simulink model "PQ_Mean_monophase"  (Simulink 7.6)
settings: Solver=ode15s  StartTime=0.0  StopTime=0.1  RelTol=1e-3
InitFcn:
  | clear all, close all
  | Arms=20;
  | T=1/60;
  | 
  | % charge de la phase C
  | R1=2;
  | 
  | % Charge R, L de la phase B
  | R=1;
  | L=0.1;
StopFcn:
  | close all
  | load PQ_PhaseC.mat
  | subplot 211
  | plot(x(1,:),x(2,:))
  | grid
  | title('Puissance active Phase C')
  | xlabel('temps')
  | 
  | subplot 212
  | plot(x(1,:),x(3,:))
  | title('Puissance réactive Phase C')
  | grid
  | xlabel('temps')
  | 
  | figure
  | 
  | load Moy_PhaseC.mat
  | subplot 211
  | plot(y(1,:),y(2,:))
  | grid
  | title('Moyenne amplitude Phase C')
  | xlabel('temps')
  | axis([0 0.1 0 1100])
  | 
  | subplot 212
  | plot(y(1,:),y(3,:))
  | title('Moyenne phase Phase C')
  | grid
  | xlabel('temps')
undefined symbols (not defined in the file or in its folder): Ts
libraries: powerlib x8, powerlib_extras x2

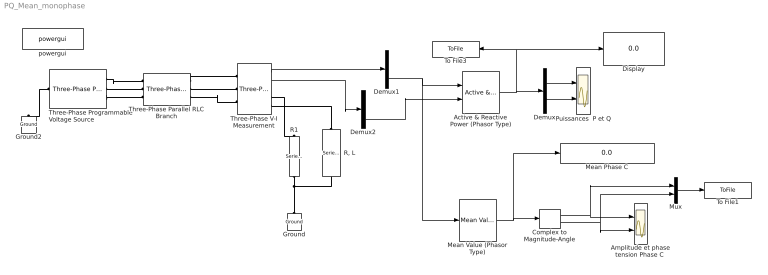
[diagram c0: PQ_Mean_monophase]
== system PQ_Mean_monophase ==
  Active & Reactive Power (Phasor Type) : powerlib_extras/Phasor Library/Active & Reactive Power (Phasor Type)  DialogController=POWERSYS.PowerSysDialog  SystemSampleTime=-1
  "Amplitude et phase tension Phase C " : Scope  NumInputPorts=2
  Complex to Magnitude-Angle : ComplexToMagnitudeAngle
  Demux : Demux  Outputs=2
  Demux1 : Demux  Outputs=3
  Demux2 : Demux  Outputs=3
  Display : Display
  Ground : powerlib/Elements/Ground  DialogController=POWERSYS.PowerSysDialog  PhysicalDomain=powersysdomain  SubClassName=unknown  LeftPortType=p1  RightPortType=p1  LConnTagsString=a
  Ground2 : powerlib/Elements/Ground  DialogController=POWERSYS.PowerSysDialog  PhysicalDomain=powersysdomain  SubClassName=unknown  LeftPortType=p1  RightPortType=p1  LConnTagsString=a
  Mean Phase C : Display
  Mean Value (Phasor Type) : powerlib_extras/Phasor Library/Mean Value (Phasor Type)  DialogController=POWERSYS.PowerSysDialog  SystemSampleTime=-1  Period=1/60
  Mux : Mux  Inputs=2
  Puissances  P et Q : Scope  NumInputPorts=2
  "R, L" : powerlib/Elements/Series RLC Branch  DialogController=POWERSYS.PowerSysDialog  PhysicalDomain=powersysdomain  SubClassName=unknown  LeftPortType=p1  RightPortType=p1  LConnTagsString=__new0  RConnTagsString=__new0  BranchType=RL  Resistance=R  Inductance=L  SetiL0=off  InitialCurrent=0  Capacitance=1e-3  Setx0=off  InitialVoltage=0  Measurements=None
  R1 : powerlib/Elements/Series RLC Branch  DialogController=POWERSYS.PowerSysDialog  PhysicalDomain=powersysdomain  SubClassName=unknown  LeftPortType=p1  RightPortType=p1  LConnTagsString=__new0  RConnTagsString=__new0  BranchType=R  Resistance=R1  Inductance=1e-3  SetiL0=off  InitialCurrent=0  Capacitance=1e-6  Setx0=off  InitialVoltage=0  Measurements=None
  Three-Phase Parallel RLC Branch : powerlib/Elements/Three-Phase Parallel RLC Branch  DialogController=POWERSYS.PowerSysDialog  PhysicalDomain=powersysdomain  SubClassName=unknown  LeftPortType=p1  RightPortType=p1  LConnTagsString=A|B|C  RConnTagsString=A|B|C  BranchType=RLC  Resistance=1  Inductance=1e-3  Capacitance=1e-6  Measurements=None
  Three-Phase Programmable Voltage Source : powerlib/Electrical Sources/Three-Phase Programmable Voltage Source  DialogController=POWERSYS.PowerSysDialog  SystemSampleTime=-1  PositiveSequence="[Arms  0 1/T]"  VariationEntity=Amplitude  VariationType=Step  VariationStep=60  VariationRate=10  VariationMagnitude=0.3  VariationFrequency=2  VariationTiming=[0.02 0.08]  VariationPhaseA=off  Amplitudes=[1 0.8 1.2 1.0]  TimeValues=[0 0.1 0.15 0.2]  HarmonicGeneration=off  HarmonicA="[3 0.2  -25 0]"  HarmonicB=[2 0.15 35 2]  Timing="[0.1  0.2]"
  Three-Phase V-I Measurement : powerlib/Measurements/Three-Phase V-I Measurement  DialogController=POWERSYS.PowerSysDialog  SystemSampleTime=-1  VoltageMeasurement=phase-to-ground  SetLabelV=off  LabelV=Vabc  Vpu=off  VpuLL=off  CurrentMeasurement=yes  SetLabelI=off  LabelI=Iabc  Ipu=off  Pbase=100e6  Vbase=500e3  OutputType=Complex  PhasorSimulation=on  PSBequivalent=0
  To File1 : ToFile  Filename=Moy_PhaseC  MatrixName=y
  To File3 : ToFile  Filename=PQ_PhaseC  MatrixName=x
  powergui : powerlib/powergui  Priority=1  SystemSampleTime=-1  SimulationMode=Phasor  SampleTime=Ts  frequency=60  SPID=off  DisableSnubberDevices=off  DisableRonSwitches=off  DisableVfSwitches=off  SwTol=0  Interpol=off  frequencyindice=60  echomessages=off  HookPort=off  DisplayEquations=off  FunctionMessages=off  EnableUseOfTLC=off  x0status=blocks  RestoreLinks=warning  ResistiveCurrentMeasurement=off  Ylog=off  Xlog=on  ShowGrid=off  save=off  variable=ZData  ZoomFFT=off  StartTime=0.0  cycles=1  DisplayStyle=1  FreqAxis=off  MaxFrequency=1000  frequencyindicesteady=1  display=off  methode=off
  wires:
  Three-Phase V-I Measurement/1 -> Demux1/1
  Three-Phase V-I Measurement/2 -> Demux2/1
  Demux1/3 -> Active & Reactive Power (Phasor Type)/1, Mean Value (Phasor Type)/1
  Demux2/3 -> Active & Reactive Power (Phasor Type)/2
  Mean Value (Phasor Type)/1 -> Complex to Magnitude-Angle/1, Mean Phase C/1
  Complex to Magnitude-Angle/1 -> "Amplitude et phase tension Phase C "/1, Mux/1
  Complex to Magnitude-Angle/2 -> "Amplitude et phase tension Phase C "/2, Mux/2
  Active & Reactive Power (Phasor Type)/1 -> Demux/1, Display/1, To File3/1
  Demux/1 -> Puissances  P et Q/1
  Demux/2 -> Puissances  P et Q/2
  Mux/1 -> To File1/1
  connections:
  R1/LConn1 -- Ground/LConn1 -- "R, L"/RConn1
  "R, L"/LConn1 -- Three-Phase V-I Measurement/RConn3
  Three-Phase V-I Measurement/RConn2 -- R1/RConn1
  Three-Phase Programmable Voltage Source/LConn1 -- Ground2/LConn1
  Three-Phase Parallel RLC Branch/RConn1 -- Three-Phase V-I Measurement/LConn1
  Three-Phase Parallel RLC Branch/RConn2 -- Three-Phase V-I Measurement/LConn2
  Three-Phase V-I Measurement/LConn3 -- Three-Phase Parallel RLC Branch/RConn3
  Three-Phase Programmable Voltage Source/RConn1 -- Three-Phase Parallel RLC Branch/LConn1
  Three-Phase Programmable Voltage Source/RConn2 -- Three-Phase Parallel RLC Branch/LConn2
  Three-Phase Programmable Voltage Source/RConn3 -- Three-Phase Parallel RLC Branch/LConn3
